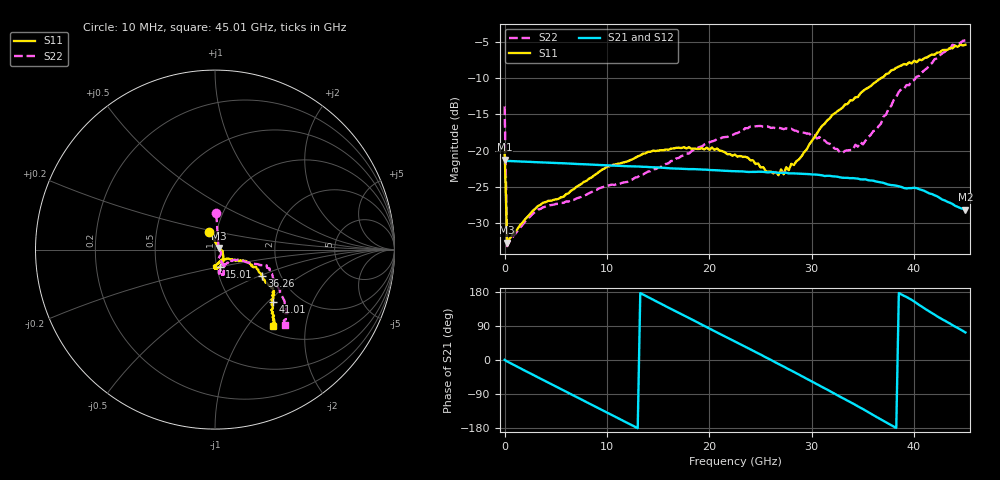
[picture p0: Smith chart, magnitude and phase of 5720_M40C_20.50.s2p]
! Device:  ADRF5720
! Description: 0.5dB LSB GaAs MMIC 6-bit Digital Attenuator
! Frequency:  0.000009 -  40 GHz
! Ports:
!	RF1	= Port 1
!	RF2	= Port 2
! Vdd:  3.3 Volt
! Vss:  -3.3 Volt
! Control:  0/3.3 Volt
! State:  20.50 dB attenuation
! Data:  The device was measured using G-S-G Probes on a matrix board.
!  Data was collected using an calibrated 4 port network analyzer.
!  The reference plane for this measurement is at the launchers.
! Note:  Analog Devices supplies this data as a sample of measured data
!  for this product.  Your particular data for this product may vary.
!  Data was taken at -40 degrees C.
!  Analog Devices reserves the right to change this data at anytime.
# GHZ S DB R 45.0
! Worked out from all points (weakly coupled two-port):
!   181 points, 10 MHz to 45.01 GHz, reference 45 ohm
!   highest |S21| = -21.26 dB at 10 MHz (marker M1); lowest = -28.2 dB at 45.01 GHz (marker M2)
!   lowest |S11| = -32.7 dB at 260 MHz (marker M3), VSWR 1.05, Z = 46.9 + j0.879 ohm
!   |S11| at or under -10 dB: start of sweep to 36.77 GHz
!   |S22| runs from -33.2 to -4.8 dB; largest |S21 - S12| = 0.00032
!   S11 on the Smith chart (normalised r, x): 10 MHz: 0.92, +0.18; 15.01 GHz: 1.04, -0.20; 36.26 GHz: 1.60, -0.51; 41.01 GHz: 1.50, -1.07; 45.01 GHz: 1.12, -1.34
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0.01  -19.85 108.7  -21.26 0.4  -21.28 0.3  -13.91 88.0
0.26  -32.73 23.9  -21.44 -3.8  -21.46 -3.9  -33.21 21.7
3.26  -27.67 -9.8  -21.62 -45.7  -21.64 -45.8  -28.18 -29.3
7.76  -24.32 -40.5  -21.89 -107.7  -21.91 -107.7  -26.22 -62.0
10.01  -22.26 -51.6  -22.05 -138.6  -22.07 -138.7  -24.88 -66.3
15.01  -20.02 -74.3  -22.34 152.2  -22.36 152.2  -22.39 -62.8
15.26  -19.95 -75.7  -22.36 148.7  -22.38 148.6  -22.25 -63.0
20.26  -19.59 -91.0  -22.70 79.6  -22.72 79.5  -18.74 -62.1
22.76  -20.86 -93.7  -22.87 45.3  -22.90 45.2  -17.58 -68.5
24.01  -21.35 -84.9  -22.96 28.3  -22.98 28.3  -16.70 -70.2
25.51  -22.83 -71.4  -22.99 7.0  -23.01 6.9  -16.70 -72.7
27.26  -23.28 -53.6  -23.07 -17.3  -23.09 -17.4  -17.05 -76.6
30.26  -18.18 -27.0  -23.31 -60.2  -23.34 -60.3  -17.89 -79.1
33.01  -14.08 -21.3  -23.76 -100.0  -23.78 -100.1  -20.32 -59.0
35.01  -11.78 -24.9  -24.00 -129.5  -24.01 -129.7  -19.15 -33.9
36.26  -10.52 -29.5  -24.27 -149.2  -24.29 -149.3  -17.20 -23.7
37.76  -8.93 -33.5  -24.77 -171.9  -24.79 -172.1  -13.84 -21.0
38.76  -8.26 -33.6  -25.03 173.0  -25.06 172.7  -11.51 -19.1
39.76  -7.97 -36.6  -25.19 158.8  -25.21 158.7  -10.40 -17.1
41.01  -7.23 -41.9  -25.58 136.2  -25.60 135.9  -8.90 -26.0
43.76  -5.88 -49.7  -27.39 91.7  -27.42 91.6  -5.39 -41.3
45.01  -5.40 -52.7  -28.18 72.7  -28.20 72.6  -4.80 -47.3
